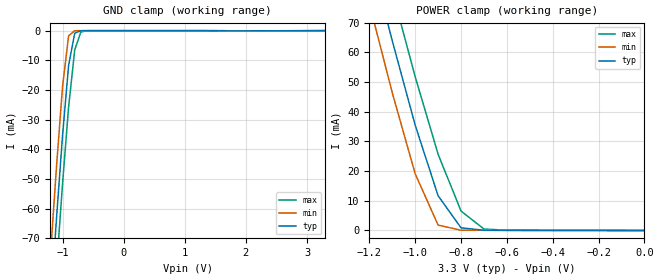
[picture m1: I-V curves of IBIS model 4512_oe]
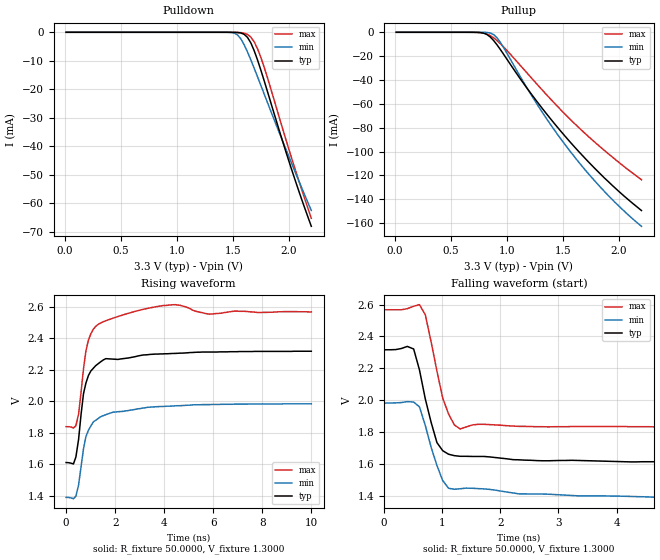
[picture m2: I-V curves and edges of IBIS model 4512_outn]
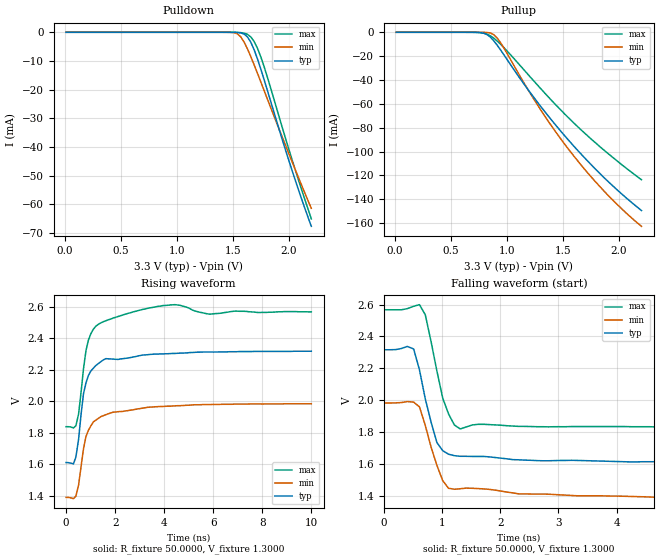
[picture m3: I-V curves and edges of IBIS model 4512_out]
| IBIS file vg4512ca4.ibs
| SEIKO EPSON Corp. 2013
[IBIS ver]   3.2
[File name]   vg4512ca4.ibs
[File Rev]   4
[Date]   Friday Jan 31 2014 02:49:07 JST
[Source]   From silicon level SPICE model.
[Notes]
[Disclaimer]   This IBIS model file is for modeling purposes only and is not
   guaranteed.
|   vg4512ca
[Component]   VG-4512CA
[Manufacturer]   SEIKO EPSON Corp.
[Package]
| variable   typ   min   max
R_pkg   0.05   0.05   0.05
L_pkg   2.00nH   2.00nH   2.00nH
C_pkg   0.50pF   0.50pF   0.50pF
[Pin]  signal_name   model_name
1   GND   GND
2   oe   4512_oe
3   GND   GND
4   out   4512_out
5   outn   4512_outn
6   vcc   POWER
| Models and submodels in the file (3): 4512_oe (Input), 4512_outn (Output_ECL), 4512_out (Output_ECL)
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|   Model 4512_oe
[Model]   4512_oe
Model_type   Input
C_comp   4.00pF  3.00pF  5.00pF
Vinl = 0.99V | VIL = VCC * 0.3
Vinh = 2.31V | VIH = VCC * 0.7
|   typ   min   max
[Temperature Range]   25.00  -40.00   85.00
[Voltage Range]   3.30V   3.00V   3.60V
[POWER Clamp Reference]   3.30V   3.00V   3.60V
[GND Clamp Reference]   0.00V   0.00V   0.00V
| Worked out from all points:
|   GND clamp passes 1 mA (typ) near -0.80 V on its own axis
|   POWER clamp passes 1 mA (typ) near -0.80 V on its own axis
[GND_clamp]
| voltage = voutput
| voltage   I(typ)   I(min)   I(max)
-3.3V     -776mA     -761mA     -790mA
-1.2V     -93.8mA    -76.4mA    -111mA
-1.1V     -63.8mA    -46.4mA    -80.6mA
-1V       -35.5mA    -19mA      -51.8mA
-900mV    -11.7mA    -1.73mA    -25.7mA
-800mV    -850uA     -21.3uA    -6.49mA
-700mV    -25uA      -5.99uA    -463uA
-600mV    -6.41uA    -5.87uA    -25.1uA
3.3V      3.29pA     24.6uA     -16.7uA
[POWER_clamp]
| voltage = vcc - voutput
| voltage   I(typ)   I(min)   I(max)
-3.3V     776mA      761mA      791mA
-1.2V     93.9mA     76.5mA     111mA
-1.1V     63.9mA     46.4mA     80.6mA
-1V       35.5mA     19.1mA     51.8mA
-900mV    11.7mA     1.81mA     25.7mA
-800mV    900uA      86uA       6.54mA
-700mV    69.3uA     61.1uA     502uA
-600mV    43.1uA     51.6uA     56.6uA
0V        3.3pA      2.99pA     3.67pA
|   Model 4512_outn
[Model]  4512_outn
Model_type Output_ECL
Polarity   Non-Inverting
Vmeas =  1.9700V
Rref =   50.0000
Vref =   1.3000V
C_comp   0.1000pF   0.1000pF   0.1000pF
[Temperature Range]   25.0000   -40.0000   85.0000
[Voltage Range]   3.3000V   3.0000V   3.6000V
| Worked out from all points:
|   rising waveform, R_fixture 50.0000, V_fixture 1.3000: 20-80 % time 451ps typ, 551ps min, 434ps max; typ from 1.61 V to 2.32 V
|   falling waveform, R_fixture 50.0000, V_fixture 1.3000: 20-80 % time 280ps typ, 311ps min, 266ps max; typ from 2.32 V to 1.61 V
[Pulldown]
|Voltage   I(typ)   I(min)   I(max)
10mV      38.99pA    48.6pA     43.7pA
1.48V     -7.291uA   -59.09uA   -6.921uA
1.54V     -75.89uA   -870.5uA   -47.06uA
1.57V     -238.1uA   -2.256mA   -121.6uA
1.6V      -699uA     -4.352mA   -308.7uA
1.63V     -1.784mA   -6.898mA   -751.4uA
1.66V     -3.733mA   -9.696mA   -1.686mA
1.69V     -6.467mA   -12.63mA   -3.344mA
1.75V     -13.34mA   -18.69mA   -8.85mA
1.81V     -20.98mA   -24.79mA   -16.12mA
2.02V     -47.63mA   -45.56mA   -43.62mA
2.2V      -68.07mA   -62.51mA   -65.28mA
[Pullup]
|Voltage   I(typ)   I(min)   I(max)
10mV      3.944pA    2.732pA    9.017pA
760mV     -244.9uA   -7.923uA   -272.9uA
820mV     -1.872mA   -148.5uA   -1.451mA
880mV     -6.961mA   -1.943mA   -4.673mA
910mV     -10.55mA   -4.666mA   -6.994mA
970mV     -18.62mA   -13.02mA   -12.46mA
1.24V     -54.76mA   -56.22mA   -40.7mA
1.39V     -72.78mA   -77.61mA   -56.16mA
1.54V     -89.52mA   -96.98mA   -70.76mA
1.72V     -108mA     -117.9mA   -86.83mA
1.9V      -124.8mA   -136.5mA   -101.5mA
2.2V      -149.4mA   -162.6mA   -123.6mA
[Ramp]
| variable   typ   min   max
dV/dt_r  0.4230/0.4502n   0.3552/0.5513n   0.4374/0.4340n
dV/dt_f  0.4242/0.2802n   0.3588/0.3113n   0.4416/0.2660n
R_load = 50.0000
[Rising Waveform]
R_fixture= 50.0000
V_fixture= 1.3000
V_fixture_min= 0.9700
V_fixture_max= 1.6300
|time   V(typ)   V(min)   V(max)
0s        1.612V     1.391V     1.839V
400ps     1.647V     1.399V     1.845V
510ps     1.759V     1.47V      1.919V
710ps     2.048V     1.699V     2.206V
810ps     2.116V     1.777V     2.32V
1.11ns    2.209V     1.869V     2.456V
1.52ns    2.262V     1.909V     2.504V
4.44ns    2.303V     1.971V     2.612V
5.86ns    2.312V     1.979V     2.552V
10ns      2.317V     1.984V     2.566V
[Falling Waveform]
R_fixture= 50.0000
V_fixture= 1.3000
V_fixture_min= 0.9700
V_fixture_max= 1.6300
|time   V(typ)   V(min)   V(max)
0s        2.317V     1.984V     2.567V
510ps     2.322V     1.99V      2.589V
610ps     2.191V     1.96V      2.599V
710ps     2.01V      1.844V     2.536V
910ps     1.737V     1.594V     2.184V
1.01ns    1.686V     1.499V     2.015V
1.11ns    1.664V     1.451V     1.916V
1.31ns    1.651V     1.448V     1.822V
4.85ns    1.617V     1.393V     1.835V
10ns      1.61V      1.386V     1.834V
|   Model 4512_out
[Model]  4512_out
Model_type Output_ECL
Polarity   Inverting
Vmeas =  1.9700V
Rref =   50.0000
Vref =   1.3000V
C_comp   0.1000pF   0.1000pF   0.1000pF
[Temperature Range]   25.0000   -40.0000   85.0000
[Voltage Range]   3.3000V   3.0000V   3.6000V
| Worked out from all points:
|   rising waveform, R_fixture 50.0000, V_fixture 1.3000: 20-80 % time 451ps typ, 551ps min, 434ps max; typ from 1.61 V to 2.32 V
|   falling waveform, R_fixture 50.0000, V_fixture 1.3000: 20-80 % time 280ps typ, 311ps min, 266ps max; typ from 2.32 V to 1.61 V
[Pulldown]
|Voltage   I(typ)   I(min)   I(max)
10mV      39.13pA    49.11pA    43.76pA
1.48V     -6.433uA   -32.52uA   -6.616uA
1.54V     -67.07uA   -540.1uA   -45uA
1.57V     -211.2uA   -1.597mA   -116.4uA
1.6V      -626.6uA   -3.432mA   -295.7uA
1.63V     -1.63mA    -5.821mA   -721.7uA
1.66V     -3.485mA   -8.529mA   -1.627mA
1.69V     -6.147mA   -11.41mA   -3.248mA
1.75V     -12.95mA   -17.41mA   -8.693mA
1.81V     -20.57mA   -23.51mA   -15.94mA
2.02V     -47.23mA   -44.34mA   -43.43mA
2.2V      -67.69mA   -61.41mA   -65.1mA
[Pullup]
|Voltage   I(typ)   I(min)   I(max)
10mV      3.908pA    2.732pA    8.818pA
760mV     -252.6uA   -7.938uA   -297.5uA
820mV     -1.916mA   -148.8uA   -1.553mA
880mV     -7.047mA   -1.945mA   -4.875mA
910mV     -10.65mA   -4.67mA    -7.229mA
970mV     -18.7mA    -13.03mA   -12.73mA
1.24V     -54.77mA   -56.23mA   -40.97mA
1.39V     -72.78mA   -77.62mA   -56.39mA
1.54V     -89.52mA   -96.99mA   -70.91mA
1.72V     -108mA     -117.9mA   -86.88mA
1.9V      -124.9mA   -136.5mA   -101.5mA
2.2V      -149.4mA   -162.6mA   -123.6mA
[Ramp]
| variable   typ   min   max
dV/dt_r  0.4248/0.4728n   0.3588/0.5797n   0.4416/0.3953n
dV/dt_f  0.4248/0.2845n   0.3588/0.3211n   0.4446/0.1981n
R_load = 50.0000
[Rising Waveform]
R_fixture= 50.0000
V_fixture= 1.3000
V_fixture_min= 0.9700
V_fixture_max= 1.6300
|time   V(typ)   V(min)   V(max)
0s        1.612V     1.391V     1.839V
400ps     1.647V     1.399V     1.845V
510ps     1.759V     1.47V      1.919V
710ps     2.048V     1.699V     2.206V
810ps     2.116V     1.777V     2.32V
1.11ns    2.209V     1.869V     2.456V
1.52ns    2.262V     1.909V     2.504V
4.44ns    2.303V     1.971V     2.612V
5.86ns    2.312V     1.979V     2.552V
10ns      2.317V     1.984V     2.566V
[Falling Waveform]
R_fixture= 50.0000
V_fixture= 1.3000
V_fixture_min= 0.9700
V_fixture_max= 1.6300
|time   V(typ)   V(min)   V(max)
0s        2.317V     1.984V     2.567V
510ps     2.322V     1.99V      2.589V
610ps     2.191V     1.96V      2.599V
710ps     2.01V      1.844V     2.536V
910ps     1.737V     1.594V     2.184V
1.01ns    1.686V     1.499V     2.015V
1.11ns    1.664V     1.451V     1.916V
1.31ns    1.651V     1.448V     1.822V
4.85ns    1.617V     1.393V     1.835V
10ns      1.61V      1.386V     1.834V
